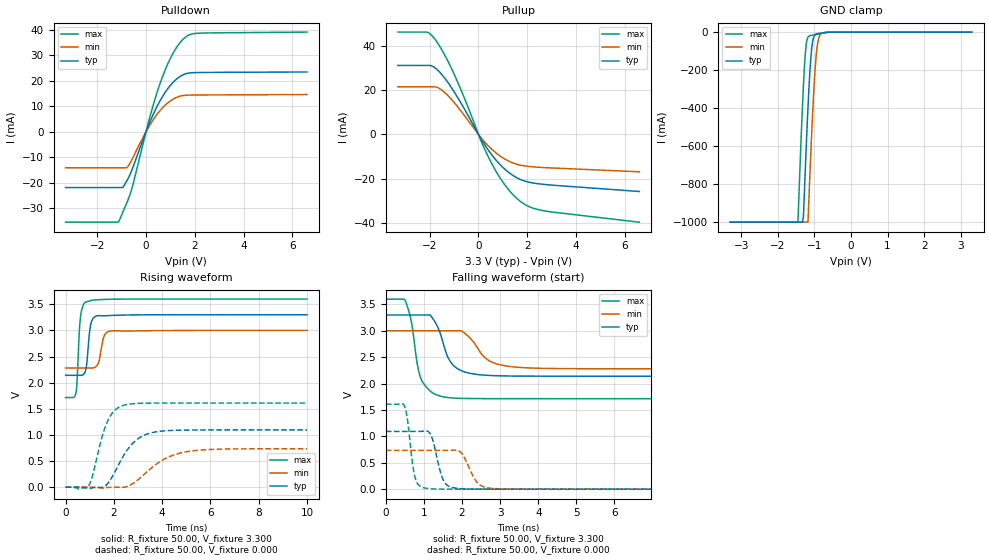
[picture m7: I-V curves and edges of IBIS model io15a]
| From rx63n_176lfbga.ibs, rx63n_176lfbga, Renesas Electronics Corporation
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[Model]   io15a
Model_type   I/O
Polarity   Non-Inverting
Enable   Active-High
Vinl  =   0.660V
Vinh  =   2.640V
Vmeas =   1.650V
Rref  =   882.000
Cref  =   30.00pF
Vref  =   3.300V
| variable   typ   min   max
C_comp   5.120pF   5.120pF   5.120pF
| variable   typ   min   max
[Temperature Range]   45.000   105.000   -40.000
| variable   typ   min   max
[Voltage Range]   3.300V   3.000V   3.600V
| variable   typ   min   max
[Pullup Reference]   3.300V   3.000V   3.600V
| variable   typ   min   max
[Pulldown Reference]   0.000V   0.000V   0.000V
| variable   typ   min   max
[POWER Clamp Reference] 3.300V   3.000V   3.600V
| variable   typ   min   max
[GND Clamp Reference]   0.000V   0.000V   0.000V
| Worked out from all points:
|   slope of the pulldown table from 0 to 0.495 V, typ, clamps not added: 46.2 ohm
|   slope of the pullup table from 0 to 0.495 V, typ, clamps not added: 58.5 ohm
|   GND clamp passes 1 mA (typ) near -0.63 V on its own axis
|   rising waveform, R_fixture 50.00, V_fixture 3.300: 20-80 % time 145ps typ, 178ps min, 127ps max; typ from 2.14 V to 3.3 V
|   rising waveform, R_fixture 50.00, V_fixture 0.000: 20-80 % time 908ps typ, 1.31ns min, 594ps max; typ from 0 V to 1.09 V
|   falling waveform, R_fixture 50.00, V_fixture 3.300: 20-80 % time 377ps typ, 515ps min, 268ps max; typ from 3.3 V to 2.14 V
|   falling waveform, R_fixture 50.00, V_fixture 0.000: 20-80 % time 228ps typ, 307ps min, 162ps max; typ from 1.09 V to 0 V
[Pulldown]
| io15a Pulldown rx631_rx63n
| Thu Mar 22 17:15:49 2012
| voltage   I(typ)   I(min)   I(max)
-3.3V     -21.93mA   -14.19mA   -35.51mA
-1.125V   -21.93mA   -14.19mA   -35.28mA
-950mV    -21.8mA    -14.19mA   -31.51mA
-725mV    -18.13mA   -13.36mA   -26.35mA
-525mV    -13.67mA   -9.89mA    -20.27mA
200mV     4.744mA    3.297mA    7.31mA
600mV     12.56mA    8.559mA    19.59mA
1.1V      19.27mA    12.7mA     30.64mA
1.375V    21.53mA    13.87mA    34.7mA
1.6V      22.62mA    14.25mA    36.96mA
2.2V      23.2mA     14.39mA    38.63mA
6.6V      23.41mA    14.56mA    39.05mA
[Pullup]
| io15a Pullup rx631_rx63n
| Thu Mar 22 17:15:49 2012
| voltage   I(typ)   I(min)   I(max)
-3.3V     31.13mA    21.49mA    46.19mA
-2.1V     31.13mA    21.49mA    46.14mA
-1.75V    29.8mA     21.42mA    42.5mA
-1.425V   26mA       19.28mA    36.71mA
-950mV    18.45mA    13.76mA    26.08mA
100mV     -1.895mA   -1.397mA   -2.764mA
550mV     -9.266mA   -6.744mA   -13.24mA
1.1V      -15.88mA   -11.28mA   -23.06mA
1.7V      -20.25mA   -13.85mA   -30.09mA
2.1V      -21.66mA   -14.51mA   -32.76mA
2.7V      -22.61mA   -15mA      -34.53mA
6.6V      -25.8mA    -16.9mA    -39.66mA
[GND Clamp]
| io15a GNDClamp rx631_rx63n
| Thu Mar 22 17:15:49 2012
| voltage   I(typ)   I(min)   I(max)
-3.3V     -1A        -1A        -1A
-1.45V    -1A        -1A        -999.2mA
-1.325V   -1A        -1A        -386.1mA
-1.3V     -972.1mA   -1A        -281.8mA
-1.25V    -727.8mA   -1A        -116.6mA
-1.175V   -394.6mA   -998.6mA   -26.29mA
-1.15V    -298.1mA   -877.8mA   -21.3mA
-1.075V   -88.02mA   -537.9mA   -16.82mA
-975mV    -12.93mA   -181.5mA   -13.67mA
-900mV    -7.441mA   -46.61mA   -11.4mA
-825mV    -5.358mA   -9.863mA   -8.608mA
3.3V      0A         0A         0A
[POWER Clamp]
| io15a PWRClamp rx631_rx63n
| Thu Mar 22 17:15:49 2012
| voltage   I(typ)   I(min)   I(max)
-3.3V     0A         0A         0A
0V        0A         0A         0A
3.3V      0A         0A         0A
[Ramp]
dV/dt_r   0.657/907.93p  0.440/1.31n   0.966/593.62p
dV/dt_f   0.696/375.20p  0.432/512.59p  1.131/267.85p
R_load = 50.00ohm
[Rising Waveform]
| io15a Rising-High rx631_rx63n
| Thu Mar 22 17:15:49 2012
R_fixture = 50.00
V_fixture = 3.300
V_fixture_min = 3.000
V_fixture_max = 3.600
C_fixture = 0.00pF
| Time   V(typ)   V(min)   V(max)
0s        2.14V      2.28V      1.714V
425ps     2.14V      2.28V      1.794V
470ps     2.14V      2.28V      1.993V
615ps     2.139V     2.28V      3.249V
865ps     2.32V      2.28V      3.548V
1.04ns    3.11V      2.279V     3.57V
1.33ns    3.283V     2.348V     3.587V
1.6ns     3.279V     2.899V     3.593V
1.905ns   3.287V     2.99V      3.597V
10ns      3.3V       3V         3.6V
[Rising Waveform]
| io15a Rising-Low rx631_rx63n
| Thu Mar 22 17:15:49 2012
R_fixture = 50.00
V_fixture = 0.000
C_fixture = 0.00pF
| Time   V(typ)   V(min)   V(max)
0s        0V         0V         0V
940ps     -25mV      0V         10mV
1.71ns    50mV       -10mV      1.23V
2.005ns   259mV      -4mV       1.455V
2.365ns   573mV      -4mV       1.56V
2.79ns    842mV      70mV       1.597V
3.255ns   993mV      244mV      1.606V
4.03ns    1.074V     521mV      1.609V
4.825ns   1.09V      660mV      1.609V
10ns      1.094V     734mV      1.609V
[Falling Waveform]
| io15a Falling-High rx631_rx63n
| Thu Mar 22 17:15:49 2012
R_fixture = 50.00
V_fixture = 3.300
V_fixture_min = 3.000
V_fixture_max = 3.600
C_fixture = 0.00pF
| Time   V(typ)   V(min)   V(max)
0s        3.3V       3V         3.6V
495ps     3.3V       3V         3.591V
660ps     3.3V       3V         3.204V
910ps     3.3V       3V         2.115V
1.165ns   3.295V     3V         1.858V
1.45ns    2.902V     3V         1.759V
1.75ns    2.363V     3V         1.728V
2.365ns   2.176V     2.721V     1.716V
3.485ns   2.143V     2.308V     1.715V
10ns      2.14V      2.28V      1.714V
[Falling Waveform]
| io15a Falling-Low rx631_rx63n
| Thu Mar 22 17:15:49 2012
R_fixture = 50.00
V_fixture = 0.000
C_fixture = 0.00pF
| Time   V(typ)   V(min)   V(max)
0s        1.094V     734mV      1.609V
485ps     1.094V     734mV      1.578V
755ps     1.094V     734mV      255mV
1.005ns   1.098V     734mV      24mV
1.2ns     994mV      734mV      7mV
1.52ns    155mV      734mV      1mV
1.83ns    19mV       741mV      0V
2.41ns    1mV        117mV      0V
2.725ns   0V         19mV       0V
10ns      0V         0V         0V
